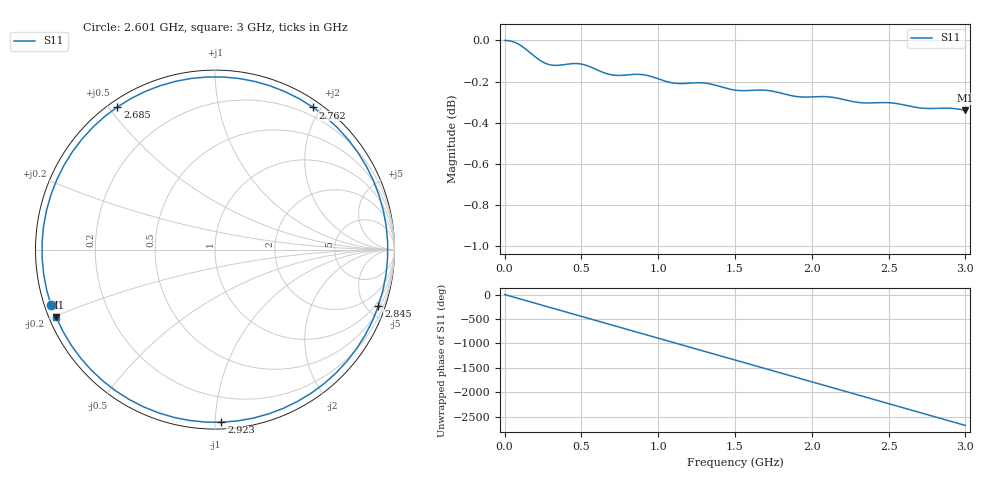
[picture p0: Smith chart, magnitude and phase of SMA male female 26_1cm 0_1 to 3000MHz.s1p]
# MHz S RI R 50.0
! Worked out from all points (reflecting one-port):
!   505 points, 100 kHz to 3 GHz, reference 50 ohm
!   lowest |S11| = -0.3 dB at 3 GHz (marker M1), VSWR 51.18, Z = 1.02 - j10.2 ohm
!   phase of S11 starts at -0 deg and turns -2677 deg over the sweep
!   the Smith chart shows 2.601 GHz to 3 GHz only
!   S11 on the Smith chart (normalised r, x): 2.601 GHz: 0.02, -0.17; 2.685 GHz: 0.02, +0.53; 2.762 GHz: 0.09, +1.90; 2.845 GHz: 0.69, -5.93; 2.923 GHz: 0.04, -1.04; 3 GHz: 0.02, -0.20
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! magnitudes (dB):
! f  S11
! 100 kHz  0.0
! 47.72 MHz  0.0
! 89.38 MHz  0.0
! 220.3 MHz  -0.1
! 267.9 MHz  -0.1
! 315.6 MHz  -0.1
! 375.1 MHz  -0.1
! 446.5 MHz  -0.1
! 500.1 MHz  -0.1
! 666.7 MHz  -0.2
! 750.1 MHz  -0.2
! 904.8 MHz  -0.2
! 1.125 GHz  -0.2
! 1.304 GHz  -0.2
! 1.5 GHz  -0.2
! 1.708 GHz  -0.2
! 1.875 GHz  -0.3
! 2.113 GHz  -0.3
! 2.25 GHz  -0.3
! 2.339 GHz  -0.3
! 2.512 GHz  -0.3
! 2.601 GHz  -0.3
! 2.625 GHz  -0.3
! 2.685 GHz  -0.3
! 2.762 GHz  -0.3
! 2.845 GHz  -0.3
! 2.923 GHz  -0.3
! 3 GHz  -0.3
